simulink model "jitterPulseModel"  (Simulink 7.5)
settings: Solver=VariableStepDiscrete  StartTime=0.0  StopTime=10.0  RelTol=1e-3

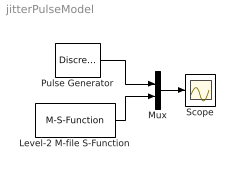
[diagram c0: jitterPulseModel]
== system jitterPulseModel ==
  Level-2 M-file S-Function : M-S-Function  FunctionName=jitterPulseSfun  Parameters=nomp,adw,ival  mask(Pulse with Jitter){nomp=2, adw=0.49, ival=1}
      mask prompts: nomp "Nominal period"; adw "Advance/Delay window"; ival "Initial value"
      mask help: Outputs a pulse whose rise/fall is centred around the specified nominal period, but which actually rises/falls before/after the nominal time based on the specified advance/delay window. A nominal 50% duty cycle is assumed, hence the advance/delay can be at most 25% of the nominal period. The initial output may be 0 or 1.
  Mux : Mux  Inputs=2
  Pulse Generator : DiscretePulseGenerator  PulseType=Time based  Amplitude=1  Period=2  PulseWidth=50  PhaseDelay=0  SampleTime=1
  Scope : Scope
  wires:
  Pulse Generator/1 -> Mux/1
  Level-2 M-file S-Function/1 -> Mux/2
  Mux/1 -> Scope/1
